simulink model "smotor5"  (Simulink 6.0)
settings: Solver=ode5  SolverMode=SingleTasking  StartTime=0.0  StopTime=5  FixedStep=0.001  RelTol=1e-3  AbsTol=1e-6
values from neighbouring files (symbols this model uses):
  bm = 3*10^(-6)    (= 3e-06)    [initmot.m]
  Jm = 30*10^(-6)    (= 3e-05)    [initmot.m]
  Kb = 60*10^(-3)    (= 0.06)    [initmot.m]
  Kt = 17*10^(-3)    (= 0.017)    [initmot.m]
  La = 8.6*10^(-3)    (= 0.0086)    [initmot.m]
  Ra = 3.2    [initmot.m]

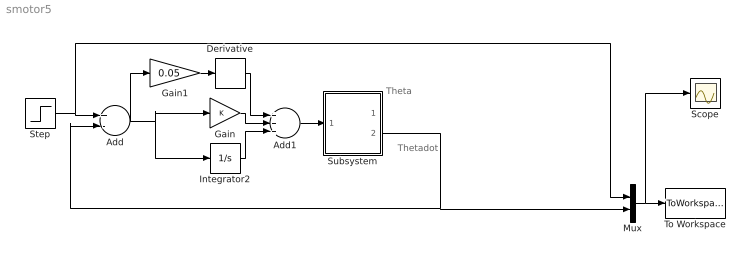
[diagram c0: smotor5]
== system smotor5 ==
  note: Theta
  note: Thetadot
  Add : Sum  Inputs=+-  OutScaling=2^-10
  Add1 : Sum  Inputs=+++  OutScaling=2^-10
  Derivative : Derivative  LinearizePole=Inf
  Gain : Gain
  Gain1 : Gain  Gain=0.05
  Integrator2 : Integrator
  Mux : Mux  Inputs=2
  Scope : Scope
  Step : Step  SampleTime=0.001
  Subsystem : Subsystem  PropExecContextAcrossSSBoundary=on
  To Workspace : ToWorkspace  VariableName=simout  SampleTime=-1  SaveFormat=Structure
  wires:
  Mux/1 -> To Workspace/1, Scope/1
  Step/1 -> Add/1, Mux/1
  Add1/1 -> Subsystem/1(In1)
  Add/1 -> Gain/1, Integrator2/1, Gain1/1
  Integrator2/1 -> Add1/3
  Gain/1 -> Add1/2
  Derivative/1 -> Add1/1
  Subsystem/2(Out2) -> Mux/2, Add/2
  Gain1/1 -> Derivative/1

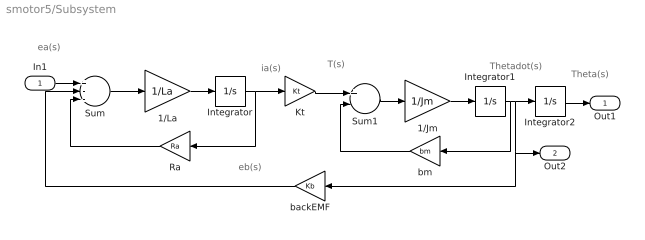
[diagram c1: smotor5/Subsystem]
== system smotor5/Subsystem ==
  note: T(s)
  note: Theta(s)
  note: Thetadot(s)
  note: ea(s)
  note: eb(s)
  note: ia(s)
  In1 : Inport  LatchInput=off
  1/Jm : Gain  Gain=1/Jm
  1/La : Gain  Gain=1/La
  Integrator : Integrator
  Integrator1 : Integrator
  Integrator2 : Integrator
  Kt : Gain  Gain=Kt
  Ra : Gain  Orientation=left  Gain=Ra
  Sum : Sum  Inputs=+--
  Sum1 : Sum  Inputs=+-
  backEMF : Gain  Orientation=left  Gain=Kb
  bm : Gain  Orientation=left  Gain=bm
  Out1 : Outport
  Out2 : Outport  Port=2
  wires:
  backEMF/1 -> Sum/2
  Kt/1 -> Sum1/1
  bm/1 -> Sum1/2
  Integrator1/1 -> backEMF/1, Out2/1, Integrator2/1, bm/1
  1/Jm/1 -> Integrator1/1
  Sum1/1 -> 1/Jm/1
  1/La/1 -> Integrator/1
  Sum/1 -> 1/La/1
  Ra/1 -> Sum/3
  Integrator/1 -> Ra/1, Kt/1
  In1/1 -> Sum/1
  Integrator2/1 -> Out1/1
